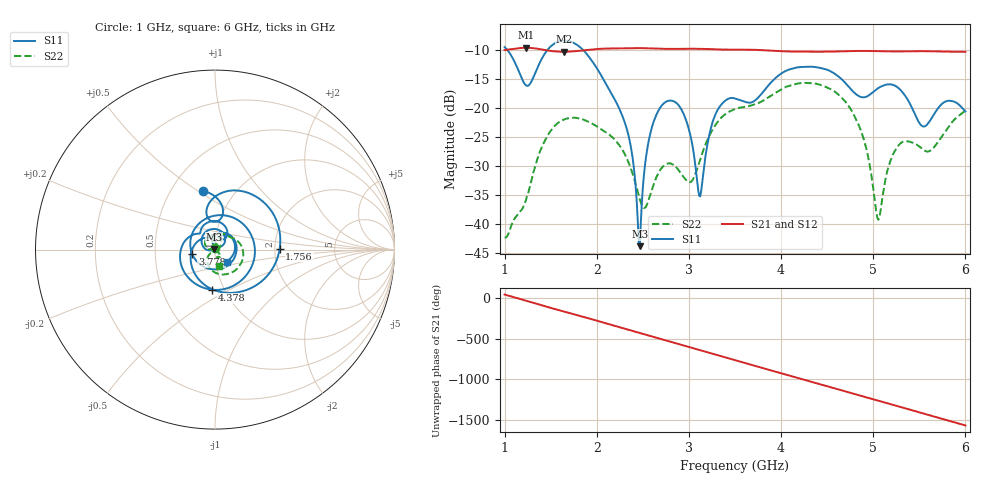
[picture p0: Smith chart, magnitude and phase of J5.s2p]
!Agilent Technologies,E8364B,MY43040528,A.07.50.67
!Agilent E8364B: A.07.50.67
!Date: Sunday, March 01, 2026 18:23:50
!Correction: S11(Full 2 Port(1,2))
!S21(Full 2 Port(1,2))
!S12(Full 2 Port(1,2))
!S22(Full 2 Port(1,2))
!S2P File: Measurements: S11, S21, S12, S22:
# Hz S  dB  R 50
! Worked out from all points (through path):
!   451 points, 1 GHz to 6 GHz, reference 50 ohm
!   highest |S21| = -9.64 dB at 1.233 GHz (marker M1); lowest = -10.3 dB at 1.644 GHz (marker M2)
!   group delay of S21, straight-line fit = 897 ps
!   lowest |S11| = -43.9 dB at 2.467 GHz (marker M3), VSWR 1.01, Z = 49.4 + j0.278 ohm
!   |S11| at or under -10 dB: 1.028 GHz to 1.467 GHz (438.4 MHz wide, 35.1 % of centre); 1.85 GHz to end of sweep
!   |S22| runs from -42.4 to -15.7 dB; largest |S21 - S12| = 0.0014
!   S11 on the Smith chart (normalised r, x): 1 GHz: 0.71, +0.52; 1.756 GHz: 2.13, +0.03; 3.778 GHz: 0.77, -0.04; 4.378 GHz: 0.88, -0.41; 6 GHz: 1.13, -0.15
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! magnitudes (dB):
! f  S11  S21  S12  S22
! 1 GHz  -9.5  -10.0  -10.1  -42.4
! 1.233 GHz  -16.1  -9.6  -9.7  -35.9
! 1.422 GHz  -11.0  -10.0  -10.0  -26.1
! 1.644 GHz  -8.4  -10.3  -10.4  -22.0
! 1.756 GHz  -8.9  -10.3  -10.3  -21.7
! 1.844 GHz  -9.9  -10.1  -10.1  -22.0
! 2.311 GHz  -22.9  -9.7  -9.8  -28.2
! 2.467 GHz  -43.9  -9.7  -9.7  -35.7
! 2.544 GHz  -27.4  -9.7  -9.8  -36.7
! 2.667 GHz  -20.6  -9.8  -9.8  -31.3
! 2.922 GHz  -20.4  -9.8  -9.9  -31.5
! 3.122 GHz  -35.3  -9.8  -9.9  -28.9
! 3.278 GHz  -21.5  -9.9  -9.9  -23.2
! 3.5 GHz  -18.4  -10.0  -10.0  -20.2
! 3.778 GHz  -17.8  -10.0  -10.1  -19.0
! 4.344 GHz  -12.9  -10.3  -10.4  -15.8
! 4.378 GHz  -13.0  -10.3  -10.4  -15.8
! 4.811 GHz  -17.6  -10.2  -10.2  -21.9
! 5.056 GHz  -16.6  -10.2  -10.3  -39.3
! 5.167 GHz  -16.0  -10.3  -10.3  -30.1
! 5.533 GHz  -23.2  -10.2  -10.3  -27.1
! 6 GHz  -20.6  -10.3  -10.4  -20.5
